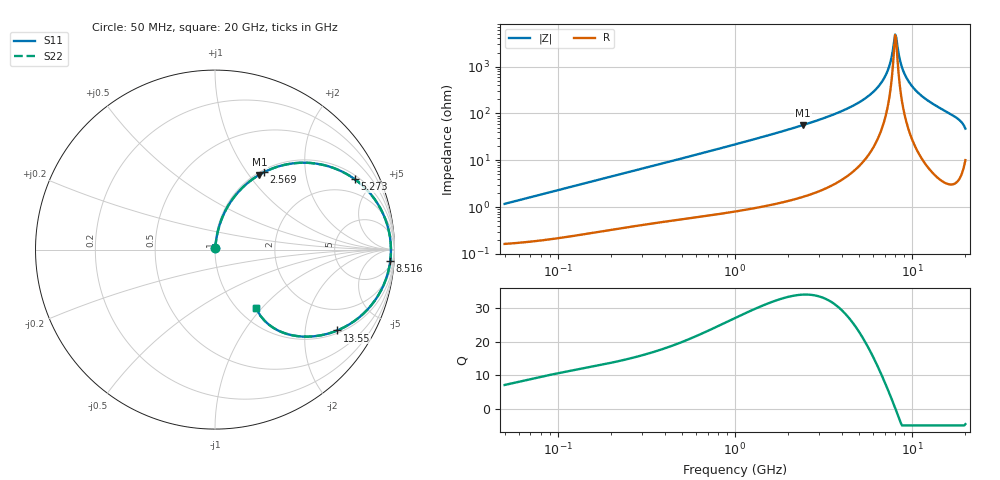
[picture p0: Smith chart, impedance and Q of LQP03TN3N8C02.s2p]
!Murata Part Number: LQP03TN3N8C02
!These Parameters are Measured in Series Mode Connection
!  o--[Z]--o
!Port1  Port2
!  o-------o
!Freq. Start=50[MHz] Stop=20[GHz], 401[Steps]
# Hz S RI R 50
!Freq.(Hz) S11(Real) S11(Imag) S21(Real) S21(Imag) S12(Real) S12(Imag) S22(Real) S22(Imag)
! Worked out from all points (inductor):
!   401 points, 50 MHz to 20 GHz, reference 50 ohm
!   read as one part in series: L = 3.68 nH near 51.52 MHz
!   highest Q = 34.1 at 2.42 GHz (marker M1), where L = 3.7 nH
!   self-resonance near 8.021 GHz
!   S11 on the Smith chart (normalised r, x): 50 MHz: 1.00, +0.02; 2.569 GHz: 1.04, +1.21; 5.273 GHz: 1.18, +3.87; 8.516 GHz: 9, -28; 13.55 GHz: 1.09, -2.96; 20 GHz: 1.20, -0.92
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5e7  0.00176 0.0115  0.9982 -0.0115  0.9982 -0.0115  0.00176 0.0115
1.364002e8  0.00352 0.0307  0.9965 -0.0307  0.9965 -0.0307  0.00352 0.0307
3.721004e8  0.0112 0.0804  0.9888 -0.0804  0.9888 -0.0804  0.0112 0.0804
1e9  0.0521 0.2045  0.9479 -0.2045  0.9479 -0.2045  0.0521 0.2045
2.419936e9  0.247 0.4168  0.753 -0.4168  0.753 -0.4168  0.247 0.4168
2.569357e9  0.2738 0.4315  0.7262 -0.4315  0.7262 -0.4315  0.2738 0.4315
2.728004e9  0.3031 0.4451  0.6969 -0.4451  0.6969 -0.4451  0.3031 0.4451
3.967106e9  0.5471 0.4812  0.4529 -0.4812  0.4529 -0.4812  0.5471 0.4812
5.273168e9  0.7786 0.3922  0.2214 -0.3922  0.2214 -0.3922  0.7786 0.3922
6.601595e9  0.9287 0.2161  0.0713 -0.2161  0.0713 -0.2161  0.9287 0.2161
7.114996e9  0.9595 0.1389  0.0405 -0.1389  0.0405 -0.1389  0.9595 0.1389
7.442007e9  0.9717 0.0897  0.0283 -0.0897  0.0283 -0.0897  0.9717 0.0897
7.901521e9  0.9798 0.0219  0.0202 -0.0219  0.0202 -0.0219  0.9798 0.0219
8.020766e9  0.9804 0.00478  0.0196 -0.00478  0.0196 -0.00478  0.9804 0.00478
8.264682e9  0.9797 -0.0296  0.0203 0.0296  0.0203 0.0296  0.9797 -0.0296
8.516016e9  0.9765 -0.0638  0.0235 0.0638  0.0235 0.0638  0.9765 -0.0638
9.041845e9  0.963 -0.1312  0.037 0.1312  0.037 0.1312  0.963 -0.1312
9.892087e9  0.9258 -0.2262  0.0742 0.2262  0.0742 0.2262  0.9258 -0.2262
1.131968e10  0.8379 -0.3462  0.1621 0.3462  0.1621 0.3462  0.8379 -0.3462
1.354865e10  0.6816 -0.4504  0.3184 0.4504  0.3184 0.4504  0.6816 -0.4504
1.747767e10  0.4215 -0.4753  0.5785 0.4753  0.5785 0.4753  0.4215 -0.4753
2e10  0.2276 -0.3244  0.7724 0.3244  0.7724 0.3244  0.2276 -0.3244
